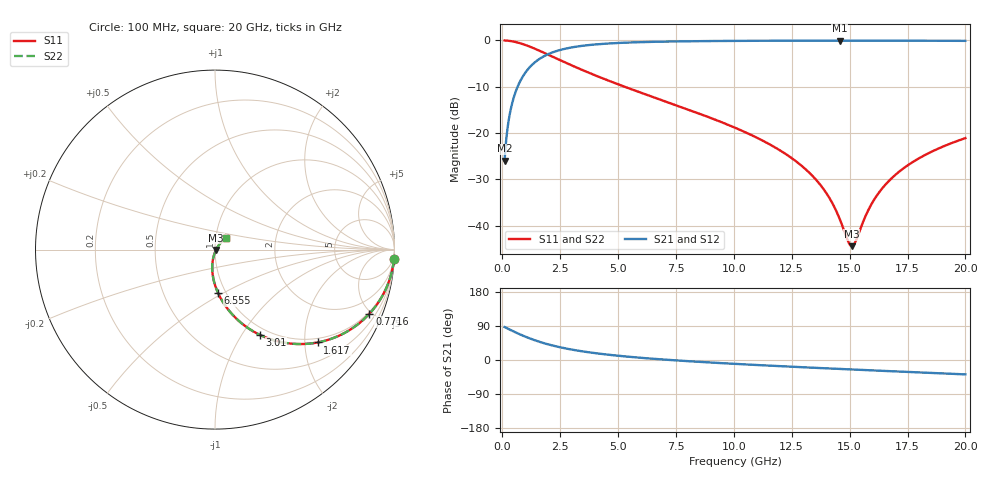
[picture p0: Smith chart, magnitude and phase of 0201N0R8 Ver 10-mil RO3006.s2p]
# GHz S MA R 50
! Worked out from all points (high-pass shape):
!   1601 points, 100 MHz to 20 GHz, reference 50 ohm
!   highest |S21| = -0.06 dB at 14.56 GHz (marker M1); lowest = -26.0 dB at 100 MHz (marker M2)
!   |S21| within 3 dB of the highest: 1.945 GHz to end of sweep
!   lowest |S11| = -44.4 dB at 15.1 GHz (marker M3), VSWR 1.01, Z = 50.5 - j0.256 ohm
!   |S11| at or under -10 dB: 5.282 GHz to end of sweep
!   |S22| runs from -44.4 to 0.0 dB; largest |S21 - S12| = 0
!   S11 on the Smith chart (normalised r, x): 100 MHz: 1, -38; 771.6 MHz: 0.90, -4.86; 1.617 GHz: 0.90, -2.30; 3.01 GHz: 0.90, -1.20; 6.555 GHz: 0.92, -0.47; 20 GHz: 1.12, +0.15
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0.1  0.9987 -3.0  0.05024 86.9  0.05024 86.9  0.9987 -3.0
0.2616875  0.9914 -7.9  0.1305 82.0  0.1305 82.0  0.9914 -7.9
0.373625  0.9827 -11.3  0.1848 78.7  0.1848 78.7  0.9827 -11.3
0.771625  0.9316 -22.5  0.3624 67.4  0.3624 67.4  0.9316 -22.5
1.617375  0.7716 -42.1  0.6342 47.8  0.6342 47.8  0.7716 -42.1
3.010375  0.5359 -62.3  0.8413 27.4  0.8413 27.4  0.5359 -62.3
3.420812  0.4836 -66.5  0.8721 23.2  0.8721 23.2  0.4836 -66.5
4.751625  0.3548 -76.6  0.9311 12.8  0.9311 12.8  0.3548 -76.6
6.555063  0.2426 -85.9  0.9657 3.1  0.9657 3.1  0.2426 -85.9
6.741625  0.2335 -86.7  0.9679 2.2  0.9679 2.2  0.2335 -86.7
10.05  0.1142 -97.7  0.9882 -10.2  0.9882 -10.2  0.1142 -97.7
12.01512  0.06454 -101.5  0.9922 -16.3  0.9922 -16.3  0.06454 -101.5
13.37081  0.03502 -100.9  0.9934 -20.2  0.9934 -20.2  0.03502 -100.9
14.04244  0.02156 -96.5  0.9936 -22.1  0.9936 -22.1  0.02156 -96.5
14.56481  0.01193 -83.9  0.9937 -23.6  0.9937 -23.6  0.01193 -83.9
14.9255  0.006851 -53.7  0.9936 -24.6  0.9936 -24.6  0.006851 -53.7
15.09962  0.006014 -24.9  0.9936 -25.0  0.9936 -25.0  0.006014 -24.9
15.26131  0.006792 1.7  0.9936 -25.5  0.9936 -25.5  0.006792 1.7
15.95781  0.01733 41.8  0.9933 -27.4  0.9933 -27.4  0.01733 41.8
16.69162  0.03033 48.7  0.9928 -29.3  0.9928 -29.3  0.03033 48.7
18.05975  0.05453 50.2  0.9915 -32.9  0.9915 -32.9  0.05453 50.2
20  0.08819 47.6  0.9888 -38.0  0.9888 -38.0  0.08819 47.6
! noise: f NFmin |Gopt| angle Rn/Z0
0.1  0.001043  0.9645  1.045  0.00665
2.301  0.00537  0.8272  4.745  0.006524
4.515  0.00829  0.7848  8.258  0.007875
6.729  0.01081  0.7578  11.8  0.008938
8.943  0.01311  0.7381  15.34  0.009844
11.14  0.01526  0.723  18.84  0.01064
13.36  0.01734  0.7107  22.33  0.01138
15.57  0.01935  0.7009  25.78  0.01206
17.79  0.02133  0.6928  29.19  0.0127
20  0.02328  0.6863  32.56  0.01331
